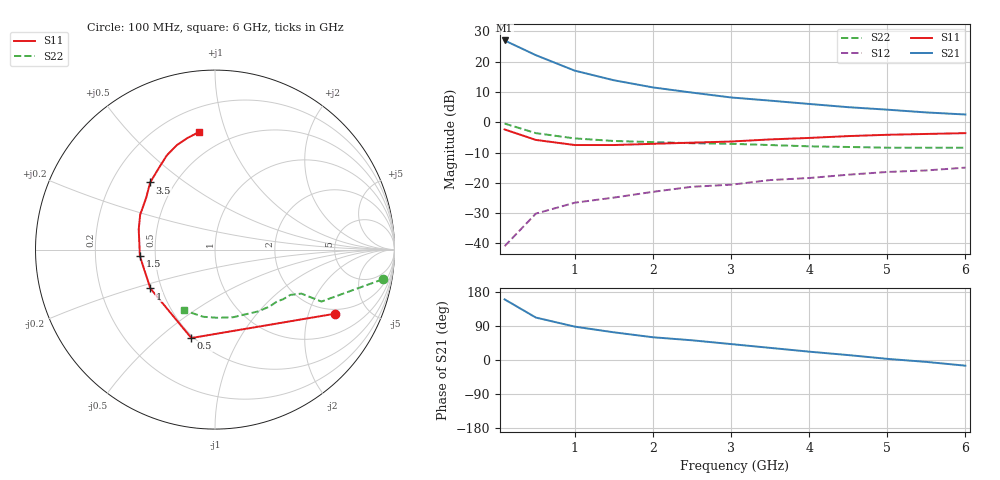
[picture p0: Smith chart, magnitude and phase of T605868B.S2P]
!AT-60586
!S-PARAMETERS at Vce=8V  Ic=10mA.  LAST UPDATED 07-21-92
# ghz s ma r 50
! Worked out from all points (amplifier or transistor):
!   13 points, 100 MHz to 6 GHz, reference 50 ohm
!   highest |S21| = 27.0 dB at 100 MHz (marker M1)
!   |S21| within 3 dB of that: start of sweep to 347 MHz
!   unconditionally stable (mu >= 1): 1.297 GHz to 4.836 GHz
!   at 1 GHz: K = 0.89, MSG = 21.8 dB, |S12| = -26.6 dB
!   at 3 GHz: K = 1.21, MAG = 11.6 dB, |S12| = -20.6 dB
!   at 6 GHz: K = 0.92, MSG = 8.8 dB, |S12| = -15.0 dB
!   S11 on the Smith chart (normalised r, x): 100 MHz: 1.79, -3.03; 500 MHz: 0.49, -0.65; 1 GHz: 0.43, -0.23; 1.5 GHz: 0.41, -0.04; 3.5 GHz: 0.37, +0.38; 6 GHz: 0.35, +0.81
0.1  0.76 -28.0  22.34 160.0  0.009 76.0  0.95 -10.0
0.5  0.51 -105.0  12.77 112.0  0.031 49.0  0.66 -26.0
1  0.42 -149.0  7.08 88.0  0.047 48.0  0.54 -27.0
1.5  0.42 -175.0  4.92 73.0  0.057 50.0  0.49 -31.0
2  0.44 165.0  3.75 60.0  0.071 51.0  0.47 -36.0
2.5  0.46 155.0  3.08 52.0  0.086 53.0  0.45 -40.0
3  0.48 143.0  2.56 42.0  0.093 48.0  0.44 -46.0
3.5  0.52 134.0  2.27 32.0  0.111 46.0  0.42 -55.0
4  0.55 125.0  2 22.0  0.12 44.0  0.4 -64.0
4.5  0.59 117.0  1.77 13.0  0.136 41.0  0.39 -75.0
5  0.62 110.0  1.61 3.0  0.151 36.0  0.38 -88.0
5.5  0.64 104.0  1.45 -5.0  0.16 34.0  0.38 -100.0
6  0.66 98.0  1.34 -15.0  0.178 30.0  0.38 -117.0
